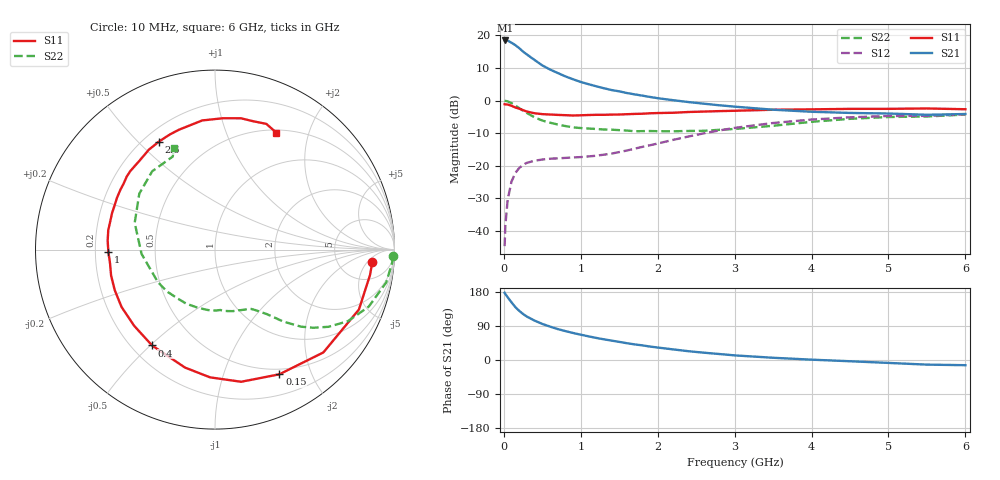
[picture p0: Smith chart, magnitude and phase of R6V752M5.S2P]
! SIEMENS Small Signal Semiconductors
! BFR193
! Si NPN RF Bipolar Junction Transistor in SOT23
! VCE = 0.75 V  IC = 2.5 mA
! Common Emitter S-Parameters:  May  1996
# GHz  S  MA  R  50
!  f  S11  S21  S12  S22
! GHz  MAG  ANG  MAG  ANG  MAG  ANG  MAG  ANG
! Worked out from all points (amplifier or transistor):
!   36 points, 10 MHz to 6 GHz, reference 50 ohm
!   highest |S21| = 18.5 dB at 20 MHz (marker M1)
!   |S21| within 3 dB of that: start of sweep to 229.9 MHz
!   unconditionally stable (mu >= 1): 1.058 GHz to 2.274 GHz; 5.386 GHz to end of sweep
!   at 250 MHz: K = 0.28, MSG = 17.4 dB, |S12| = -19.7 dB
!   at 1.4 GHz: K = 1.13, MAG = 7.6 dB, |S12| = -16.3 dB
!   at 6 GHz: K = 1.00, MAG = -0.4 dB, |S12| = -4.2 dB
!   S11 on the Smith chart (normalised r, x): 10 MHz: 11, -7; 150 MHz: 0.43, -1.55; 400 MHz: 0.28, -0.51; 1 GHz: 0.25, -0.01; 2.6 GHz: 0.26, +0.58; 6 GHz: 0.53, +1.52
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0.01  0.879 -4.6  8.29 177.4  0.0058 87.4  0.9947 -2.1
0.02  0.8753 -9.3  8.387 174.0  0.0122 83.8  0.9894 -4.3
0.05  0.8686 -22.6  8.342 165.5  0.0301 77.2  0.9718 -10.8
0.1  0.8323 -43.5  7.736 152.1  0.0573 67.0  0.914 -20.3
0.15  0.7819 -62.7  7.104 139.4  0.0773 58.0  0.8411 -28.3
0.2  0.7507 -78.8  6.391 129.7  0.0922 50.9  0.7652 -34.2
0.25  0.7124 -92.2  5.651 121.4  0.103 45.1  0.6996 -38.5
0.3  0.6781 -104.3  5.107 114.5  0.1106 41.4  0.6444 -41.8
0.4  0.6388 -123.3  4.199 103.9  0.119 35.9  0.5527 -46.5
0.5  0.619 -136.6  3.471 95.2  0.1243 33.0  0.4936 -49.3
0.6  0.611 -148.4  3.001 88.1  0.1279 31.2  0.4574 -51.5
0.8  0.5967 -165.9  2.353 76.3  0.1316 31.8  0.4062 -56.2
1  0.5944 -178.9  1.93 66.7  0.1355 34.9  0.3786 -61.1
1.1  0.6001 175.2  1.787 62.5  0.1387 36.6  0.3721 -64.1
1.3  0.6044 164.9  1.547 54.6  0.1476 41.0  0.3595 -70.1
1.6  0.6177 152.1  1.306 44.3  0.171 47.6  0.3461 -81.0
2.2  0.6499 130.3  1.014 28.0  0.2492 52.0  0.3375 -107.2
2.6  0.6778 117.5  0.896 19.3  0.3142 49.2  0.3433 -128.3
3.5  0.7232 95.6  0.724 5.9  0.4525 34.6  0.41 -176.7
4.5  0.7457 78.9  0.646 -3.3  0.5537 16.3  0.5242 143.6
5.5  0.7566 67.8  0.605 -12.2  0.5823 -0.2  0.5695 114.4
6  0.7361 62.4  0.622 -13.7  0.6137 -5.0  0.6109 112.0
